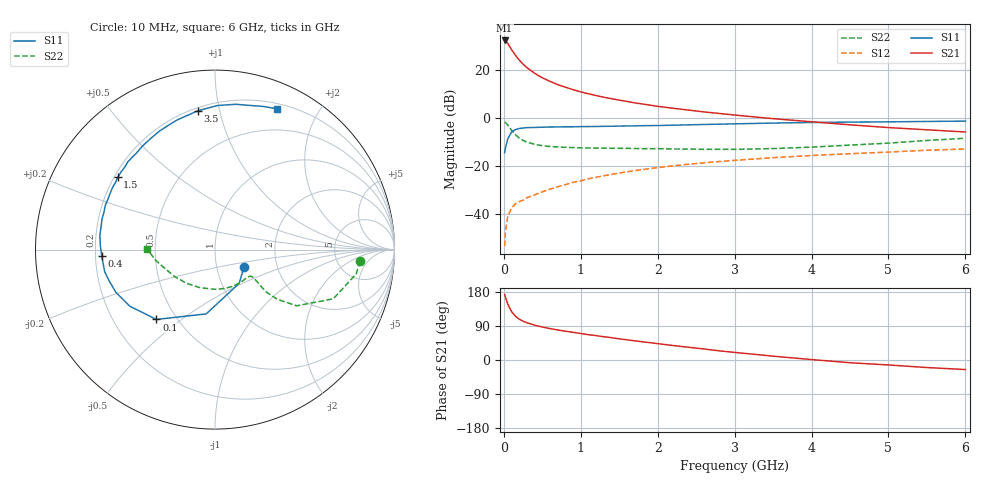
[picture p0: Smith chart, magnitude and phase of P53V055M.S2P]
! SIEMENS Small Signal Semiconductors
! BFP183
! Si NPN RF Bipolar Junction Transistor in SOT143
! VCE = 3 V  IC = 55 mA
! Common Emitter S-Parameters:  March  1996
# GHz  S  MA  R  50
!  f  S11  S21  S12  S22
! GHz  MAG  ANG  MAG  ANG  MAG  ANG  MAG  ANG
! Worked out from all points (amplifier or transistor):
!   36 points, 10 MHz to 6 GHz, reference 50 ohm
!   highest |S21| = 32.3 dB at 10 MHz (marker M1)
!   |S21| within 3 dB of that: start of sweep to 84.84 MHz
!   unconditionally stable (mu >= 1): start of sweep to 20.66 MHz; 248.2 MHz to end of sweep
!   at 250 MHz: K = 1.01, MAG = 28.0 dB, |S12| = -34.4 dB
!   at 1.4 GHz: K = 1.51, MAG = 11.6 dB, |S12| = -23.6 dB
!   at 6 GHz: K = 1.15, MAG = 1.2 dB, |S12| = -13.0 dB
!   S11 on the Smith chart (normalised r, x): 10 MHz: 1.36, -0.27; 100 MHz: 0.39, -0.41; 400 MHz: 0.23, -0.03; 1.5 GHz: 0.21, +0.32; 3.5 GHz: 0.22, +0.86; 6 GHz: 0.25, +1.50
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0.01  0.1883 -30.7  41.4 173.1  0.0021 69.1  0.8093 -4.5
0.02  0.2314 -54.4  40.77 166.5  0.0041 68.9  0.7989 -9.7
0.05  0.3616 -97.8  36.14 148.1  0.0086 67.8  0.7136 -22.6
0.1  0.5079 -130.0  26.75 127.7  0.0131 52.0  0.5527 -34.5
0.15  0.5699 -146.4  20.35 115.6  0.016 49.7  0.4464 -38.5
0.2  0.6014 -156.7  16.13 107.8  0.0179 49.2  0.3803 -39.5
0.25  0.6149 -163.5  13.26 102.3  0.0191 50.4  0.3395 -39.0
0.3  0.6268 -168.7  11.24 98.3  0.0216 52.2  0.3124 -38.0
0.4  0.6319 -176.6  8.564 91.9  0.0247 54.7  0.2811 -36.7
0.5  0.6397 177.7  6.867 87.1  0.0287 56.4  0.263 -36.2
0.6  0.6464 172.8  5.81 82.9  0.0326 59.0  0.2535 -36.3
0.7  0.6472 168.9  4.956 79.3  0.0365 60.2  0.2471 -36.8
0.9  0.6524 161.8  3.892 73.1  0.0452 61.4  0.2402 -39.1
1.1  0.6594 154.8  3.191 66.8  0.0537 61.5  0.2354 -42.5
1.5  0.6751 143.4  2.35 55.8  0.0708 59.8  0.2315 -50.8
1.8  0.689 134.8  1.954 48.1  0.0833 57.6  0.2278 -58.5
2.2  0.7052 124.6  1.59 38.2  0.0998 54.0  0.2244 -69.4
2.8  0.74 110.4  1.238 24.2  0.1229 47.9  0.2213 -88.6
3.5  0.7795 97.0  0.964 10.1  0.1478 41.1  0.2288 -112.7
4.5  0.8178 81.9  0.717 -7.2  0.179 31.1  0.2704 -146.1
5.5  0.8429 71.0  0.565 -19.9  0.2115 22.0  0.3378 -170.1
6  0.8566 66.3  0.508 -25.2  0.2248 17.0  0.3765 179.7
